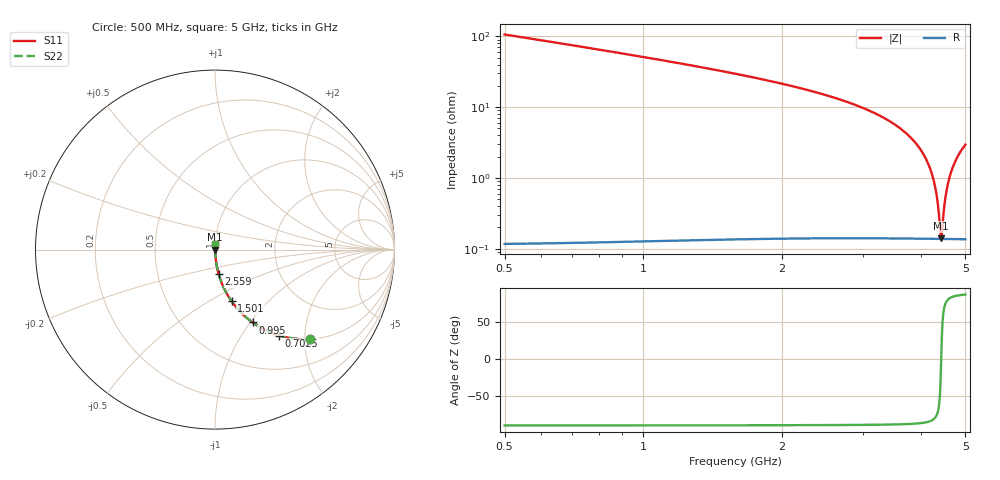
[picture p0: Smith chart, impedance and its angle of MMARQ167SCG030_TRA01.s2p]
! MMARQ167SCG030_TRA01  S-PARAMETER MODEL  ( General Type )
! Model Generated by TAIYO YUDEN Corporation (http://www.ty-top.com)
! Version 1.0
! TAIYO YUDEN Control No. 150305
! Copyright(c) 2015 TAIYO YUDEN CO.,LTD. All Rights Reserved.
! Product Description (link to TY-COMPAS)
! https://ds.yuden.co.jp/TYCOMPAS/or/detail?pn=MMARQ167SCG030BTRA01&u=M
! Products Name : Multilayer Ceramic Capacitors
! Characteristics :
!  Capacitance : 3 pF , Rated Voltage : 250V , TCC : CG / C0G
!  Case Size : 1.6 x 0.8 / 0.063 x 0.031 [mm/inch] , Thickness : 0.7 / 0.028 [mm/inch]
!  (Conditions: Temperature = 25 degC , DC Bias Current/Voltage = 0A / 0V)
! External Node Assignments :
!  1  o---| |---o  2
! GND o---------o GND
! Frequency Range : 500MHz  -  5GHz  [ 401 STEP ]
# MHz S RI R 50
! Freq[MHz].  S11 Real  S11 Imag  S21 Real  S21 Imag  S12 Real  S12 Imag  S22 Real  S22 Imag
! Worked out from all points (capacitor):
!   401 points, 500 MHz to 5 GHz, reference 50 ohm
!   read as one part in series: C = 2.96 pF near 522.5 MHz
!   lowest |Z| = 140 mohm at 4.426 GHz (marker M1)
!   series resonance near 4.431 GHz, so ESL is about 440 pH
!   S11 on the Smith chart (normalised r, x): 500 MHz: 1.00, -2.13; 702.5 MHz: 1.00, -1.49; 995 MHz: 1.00, -1.03; 1.501 GHz: 1.00, -0.63; 2.559 GHz: 1.00, -0.28; 5 GHz: 1.00, +0.06
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500  0.5303 -0.4985  0.4697 0.4985  0.4697 0.4985  0.5303 -0.4985
702.5  0.3582 -0.4787  0.6418 0.4787  0.6418 0.4787  0.3582 -0.4787
995  0.2092 -0.4055  0.7908 0.4055  0.7908 0.4055  0.2092 -0.4055
1253.75  0.1357 -0.3408  0.8643 0.3408  0.8643 0.3408  0.1357 -0.3408
1501.25  0.0924 -0.2875  0.9076 0.2875  0.9076 0.2875  0.0924 -0.2875
2007.5  0.0446 -0.2032  0.9554 0.2032  0.9554 0.2032  0.0446 -0.2032
2558.75  0.0206 -0.1371  0.9794 0.1371  0.9794 0.1371  0.0206 -0.1371
2750  0.0156 -0.1182  0.9844 0.1182  0.9844 0.1182  0.0156 -0.1182
3503.75  0.00468 -0.0572  0.9953 0.0572  0.9953 0.0572  0.00468 -0.0572
3976.25  0.00208 -0.0262  0.9979 0.0262  0.9979 0.0262  0.00208 -0.0262
4133.75  0.00167 -0.0168  0.9983 0.0168  0.9983 0.0168  0.00167 -0.0168
4257.5  0.00147 -0.00966  0.9985 0.00966  0.9985 0.00966  0.00147 -0.00966
4336.25  0.0014 -0.00522  0.9986 0.00522  0.9986 0.00522  0.0014 -0.00522
4370  0.00139 -0.00334  0.9986 0.00334  0.9986 0.00334  0.00139 -0.00334
4415  0.00138 -0.000862  0.9986 0.000862  0.9986 0.000862  0.00138 -0.000862
4426.25  0.00137 -0.000246  0.9986 0.000246  0.9986 0.000246  0.00137 -0.000246
4448.75  0.00138 0.000982  0.9986 -0.000982  0.9986 -0.000982  0.00138 0.000982
4493.75  0.00138 0.00342  0.9986 -0.00342  0.9986 -0.00342  0.00138 0.00342
4527.5  0.0014 0.00523  0.9986 -0.00523  0.9986 -0.00523  0.0014 0.00523
4628.75  0.00148 0.0106  0.9985 -0.0106  0.9985 -0.0106  0.00148 0.0106
4786.25  0.00172 0.0187  0.9983 -0.0187  0.9983 -0.0187  0.00172 0.0187
5000  0.00222 0.0293  0.9978 -0.0293  0.9978 -0.0293  0.00222 0.0293
